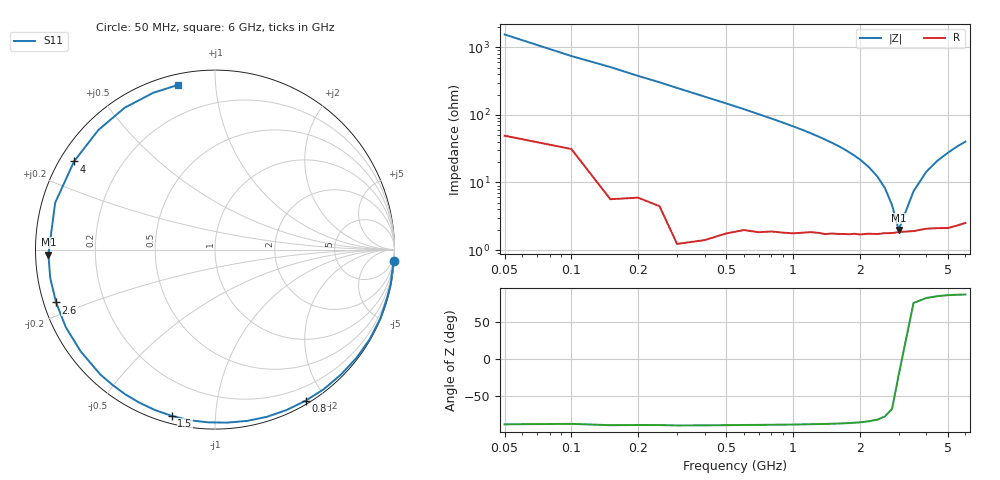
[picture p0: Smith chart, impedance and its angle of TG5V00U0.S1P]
! SIEMENS Discrete & RF Semiconductors
! BAT64
! Si Schottky Diode in SOT23
! VR = 5 V
! S-Parameters:  February  1997
# GHz  S  MA  R  50
!  f  S11
! GHz  MAG  ANG
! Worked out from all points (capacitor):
!   34 points, 50 MHz to 6 GHz, reference 50 ohm
!   read as one part to ground: C = 2.08 pF near 50 MHz
!   lowest |Z| = 1.99 ohm at 3 GHz (marker M1)
!   series resonance near 3.047 GHz, so ESL is about 1.3 nH
!   S11 on the Smith chart (normalised r, x): 50 MHz: 1, -31; 800 MHz: 0.04, -1.76; 1.5 GHz: 0.04, -0.77; 2.6 GHz: 0.04, -0.16; 4 GHz: 0.04, +0.29; 6 GHz: 0.05, +0.80
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0.05  0.998 -3.7
0.15  0.9979 -11.2
0.25  0.9953 -18.7
0.4  0.9962 -30.1
0.5  0.9928 -37.4
0.6  0.9886 -44.7
0.7  0.986 -52.0
0.8  0.9819 -59.1
0.9  0.9788 -66.0
1  0.9754 -72.8
1.1  0.971 -79.4
1.3  0.9632 -92.3
1.4  0.9611 -98.6
1.5  0.9569 -104.6
1.6  0.9544 -110.4
1.8  0.9489 -121.9
2  0.9446 -132.5
2.2  0.9392 -142.8
2.4  0.9369 -152.5
2.6  0.933 -161.6
2.8  0.9316 -170.2
3  0.9287 -178.3
3.5  0.9279 163.7
4  0.9263 148.0
4.5  0.9308 134.3
5  0.937 122.5
5.5  0.939 111.5
6  0.9405 102.5
